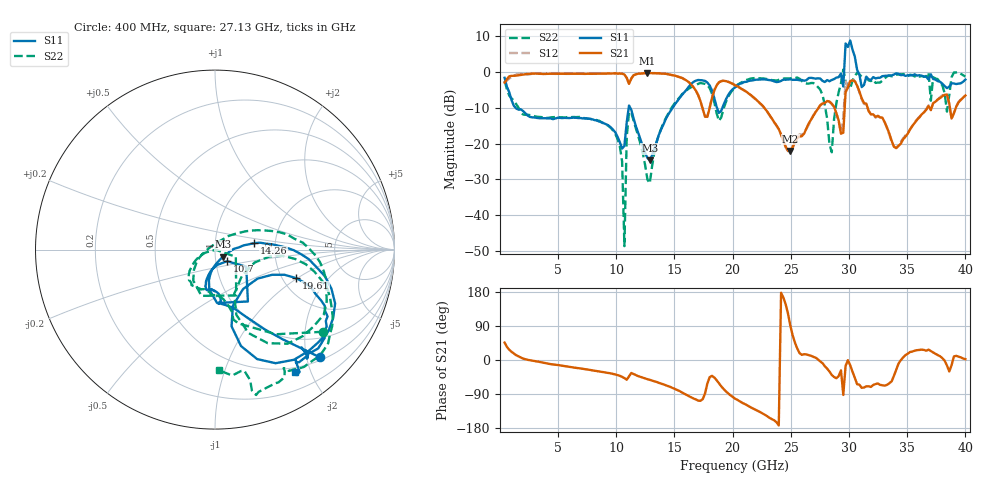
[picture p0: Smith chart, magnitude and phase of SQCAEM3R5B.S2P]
! Network Analyzer HP8722ES.07.66: Jul 25, 2000 Serial No. US39175408
! 26 Oct 2004  14:05:04
! Frequency  S11  S21  S12  S22
# HZ  S  DB R  50
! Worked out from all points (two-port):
!   201 points, 400 MHz to 40 GHz, reference 50 ohm
!   highest |S21| = -0.24 dB at 12.68 GHz (marker M1); lowest = -22.0 dB at 24.95 GHz (marker M2)
!   |S21| within 3 dB of the highest: start of sweep to 11.09 GHz; 11.1 GHz to 16.36 GHz (5.268 GHz wide, 38.4 % of centre)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
!   lowest |S11| = -24.6 dB at 12.87 GHz (marker M3), VSWR 1.13, Z = 54.4 - j4.26 ohm
!   |S11| at or under -10 dB: 1.352 GHz to 11.06 GHz (9.711 GHz wide, 156 % of centre); 11.2 GHz to 14.82 GHz (3.615 GHz wide, 27.8 % of centre); 18.65 GHz to 19.11 GHz (457.8 MHz wide, 2.42 % of centre)
!   |S22| runs from -48.7 to 0.7 dB; largest |S21 - S12| = 0.25
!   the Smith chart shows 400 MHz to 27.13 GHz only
!   S11 on the Smith chart (normalised r, x): 400 MHz: 0.57, -2.25; 10.7 GHz: 1.13, -0.15; 14.26 GHz: 1.56, +0.12; 19.61 GHz: 2.36, -0.97; 27.13 GHz: 0.44, -1.77
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4e8  -1.56 -45.8  -2.90 45.9  -3.12 50.9  -2.43 -37.3
7.132e9  -12.92 -102.6  -0.43 -23.2  -0.46 -23.6  -12.74 -124.6
1.0102e10  -18.04 -101.8  -0.38 -39.9  -0.34 -39.8  -18.64 -152.2
1.0696e10  -20.58 -43.9  -0.64 -47.8  -0.64 -47.9  -48.68 -13.2
1.1092e10  -9.31 -57.6  -3.27 -43.0  -3.29 -42.3  -11.01 -65.1
1.2676e10  -24.03 -64.6  -0.24 -50.6  -0.23 -50.5  -30.07 158.8
1.2874e10  -24.60 -41.5  -0.26 -52.4  -0.26 -52.5  -31.07 103.5
1.3666e10  -17.43 5.4  -0.29 -60.4  -0.32 -60.3  -17.44 39.3
1.426e10  -13.03 9.4  -0.45 -66.7  -0.45 -66.7  -12.82 27.7
1.9606e10  -6.41 -19.4  -2.68 -87.9  -2.65 -88.1  -6.96 -6.6
2.02e10  -4.26 -23.8  -3.68 -102.0  -3.58 -101.3  -4.12 -16.3
2.4952e10  -1.99 -49.9  -22.01 91.0  -22.07 90.8  -1.72 -68.6
2.6932e10  -1.68 -57.8  -12.20 8.4  -12.03 9.0  -3.03 -82.6
2.713e10  -1.80 -56.7  -11.13 6.1  -11.08 6.8  -3.44 -88.1
2.9506e10  -4.01 26.9  -16.94 -92.2  -12.70 -73.5  0.73 44.2
2.9704e10  8.06 -49.3  -5.62 -15.3  -2.61 -3.3  -2.60 -81.6
3.01e10  8.89 -67.2  -2.50 -13.6  -2.46 -13.6  -4.62 -22.0
3.0496e10  4.38 -80.5  -2.50 -46.9  -2.47 -45.4  -1.08 -37.0
3.0694e10  0.67 89.6  -3.76 -63.8  -3.77 -62.0  -0.16 134.7
3.1486e10  -1.25 -50.3  -8.81 -69.5  -8.94 -69.9  -1.52 -55.8
3.3466e10  -0.90 -39.7  -17.20 -61.4  -17.51 -60.3  -0.94 -44.3
4e10  -2.07 -68.3  -6.50 2.2  -6.60 3.8  -1.21 -44.7
